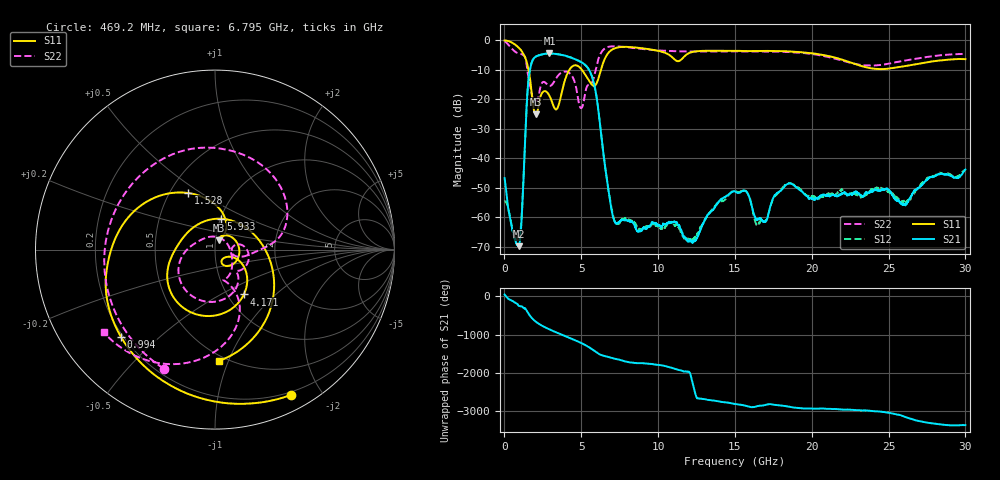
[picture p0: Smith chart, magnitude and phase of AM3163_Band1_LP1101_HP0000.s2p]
!Agilent Technologies,E8364B,MY43040894,A.07.50.67
!Agilent E8364B: A.07.50.67
!Date: Thursday, August 20, 2020 11:28:15
!Correction: S11(Full 2 Port(1,2))
!S21(Full 2 Port(1,2))
!S12(Full 2 Port(1,2))
!S22(Full 2 Port(1,2))
!S2P File: Measurements: S11, S21, S12, S22:
# Hz S  dB  R 50
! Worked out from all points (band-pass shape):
!   3201 points, 10 MHz to 30 GHz, reference 50 ohm
!   highest |S21| = -4.51 dB at 2.925 GHz (marker M1); lowest = -69.8 dB at 919.1 MHz (marker M2)
!   |S21| within 3 dB of the highest: 1.777 GHz to 5.019 GHz (3.242 GHz wide, 95.4 % of centre)
!   lowest |S11| = -25.1 dB at 2.044 GHz (marker M3), VSWR 1.12, Z = 52 + j5.33 ohm
!   |S11| at or under -10 dB: 1.564 GHz to 4.231 GHz (2.667 GHz wide, 92.1 % of centre); 5.033 GHz to 6.284 GHz (1.25 GHz wide, 22.1 % of centre)
!   |S22| runs from -23.0 to -0.4 dB; largest |S21 - S12| = 0.0061
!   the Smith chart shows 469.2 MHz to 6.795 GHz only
!   S11 on the Smith chart (normalised r, x): 469.2 MHz: 0.17, -1.64; 994 MHz: 0.19, -0.38; 1.528 GHz: 0.62, +0.44; 4.171 GHz: 1.19, -0.65; 5.933 GHz: 1.00, +0.36; 6.795 GHz: 0.46, -0.92
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1e7  -0.11 -9.0  -46.70 50.8  -54.65 -51.7  -0.41 -17.9
4.692219e8  -0.78 -62.4  -62.94 -108.7  -62.78 -108.2  -2.83 -113.4
9.190719e8  -2.53 -125.4  -69.75 117.8  -67.58 122.1  -4.53 152.2
9.940469e8  -2.91 -137.1  -68.37 110.1  -66.70 -126.4  -4.63 135.9
1.528244e9  -9.13 115.6  -15.46 -63.3  -15.46 -63.4  -11.68 0.8
2.043697e9  -25.07 66.2  -5.55 57.1  -5.56 57.1  -20.56 1.0
2.352969e9  -18.94 40.2  -4.97 -24.7  -4.96 -24.8  -15.65 5.6
2.924653e9  -18.81 -53.2  -4.51 -142.1  -4.52 -142.1  -15.49 -45.2
3.580684e9  -21.00 -26.3  -4.85 103.5  -4.88 103.5  -11.49 -70.8
4.171112e9  -10.54 -57.2  -5.61 5.6  -5.63 5.8  -10.95 -122.1
5.014581e9  -9.87 -145.1  -7.50 -142.7  -7.47 -142.7  -22.97 53.5
5.933025e9  -15.14 79.4  -17.34 -9.2  -17.39 -9.4  -10.14 -64.9
6.795238e9  -4.13 -88.1  -51.72 -146.9  -51.72 -147.2  -2.24 -143.3
7.985466e9  -2.29 179.5  -61.10 88.4  -60.43 85.3  -2.42 147.4
1.000979e10  -3.63 82.0  -62.55 5.0  -63.14 6.6  -3.47 63.9
1.231527e10  -3.93 14.5  -68.30 142.9  -67.14 170.6  -3.85 -16.4
1.5005e10  -3.62 -71.6  -51.21 61.3  -51.15 62.3  -3.81 -92.2
1.647638e10  -3.65 -107.1  -60.73 8.8  -62.23 10.0  -3.83 -128.3
2.000958e10  -4.43 163.4  -53.71 -58.2  -52.89 -59.0  -4.69 136.4
2.274617e10  -7.97 60.9  -51.62 -98.2  -51.77 -98.4  -7.98 21.3
2.500479e10  -9.66 -62.4  -50.78 -167.2  -51.40 -168.5  -7.99 -92.4
3e10  -6.44 104.7  -43.81 -132.4  -43.76 -132.8  -4.64 102.0
